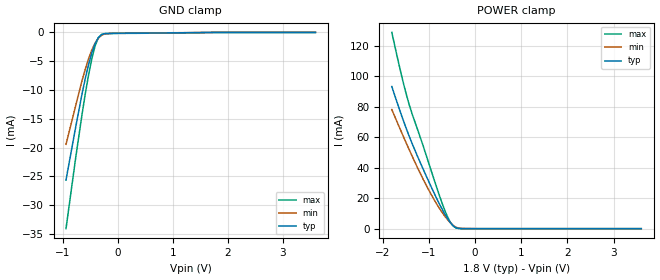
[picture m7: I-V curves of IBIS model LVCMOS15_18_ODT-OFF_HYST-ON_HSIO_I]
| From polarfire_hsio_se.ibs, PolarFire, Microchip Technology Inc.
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|   Model LVCMOS15_18_ODT-OFF_HYST-ON_HSIO_I
[Model]   LVCMOS15_18_ODT-OFF_HYST-ON_HSIO_I
Model_type   Input
Vinl =   0.525
Vinh =   0.975
|   typ   min   max
C_comp_pullup   1.335e-12   1.335e-12   1.380e-12
C_comp_pulldown  1.335e-12   1.335e-12   1.380e-12
[Model Spec]
Vinh+   0.780   NA   NA
Vinh-   0.780   NA   NA
Vinl+   0.720   NA   NA
Vinl-   0.720   NA   NA
[Temperature Range]  25C   100C   -40C
[Voltage Range]  1.8   1.71   1.89
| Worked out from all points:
|   GND clamp passes 1 mA (typ) near -0.36 V on its own axis
|   POWER clamp passes 1 mA (typ) near -0.43 V on its own axis
[GND Clamp]
| Voltage   I(typ)   I(min)   I(max)
-945mV    -25.64mA   -19.44mA   -34.09mA
-767.8mV  -16.42mA   -12.66mA   -21.74mA
-649.7mV  -10.53mA   -8.28mA    -14.04mA
-590.6mV  -7.869mA   -6.289mA   -10.5mA
-531.6mV  -5.486mA   -4.51mA    -7.275mA
-472.5mV  -3.471mA   -3.004mA   -4.488mA
-413.4mV  -1.919mA   -1.821mA   -2.303mA
-354.4mV  -899.8uA   -991.2uA   -913.4uA
-295.3mV  -390.3uA   -497.2uA   -345.4uA
-236.2mV  -211.8uA   -259.6uA   -216.3uA
-59.06mV  -146uA     -125.3uA   -182.8uA
3.6V      0A         0A         0A
[POWER Clamp]
| Voltage   I(typ)   I(min)   I(max)
-1.8V     93.14mA    78.04mA    128.6mA
-1.654V   79.85mA    67.65mA    108.7mA
-1.536V   69.63mA    59.4mA     93.76mA
-1.417V   60.1mA     51.35mA    80.64mA
-1.358V   55.64mA    47.4mA     74.99mA
-1.004V   31.09mA    25.49mA    43.29mA
-708.7mV  12.66mA    10.53mA    16.47mA
-590.6mV  6.471mA    5.78mA     7.542mA
-472.5mV  1.945mA    2.17mA     1.748mA
-354.4mV  180.5uA    381.1uA    114.2uA
-236.2mV  28.78uA    101.7uA    30.8uA
3.6V      0A         0A         0A
